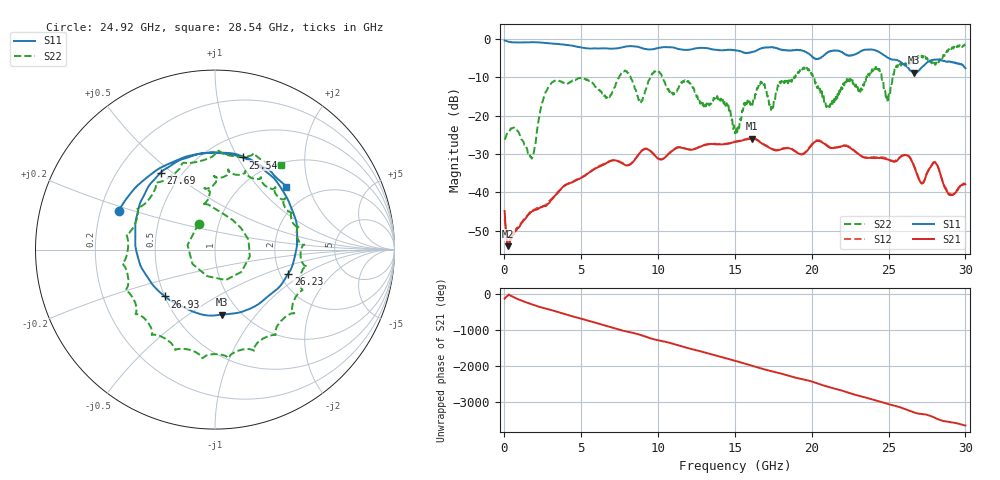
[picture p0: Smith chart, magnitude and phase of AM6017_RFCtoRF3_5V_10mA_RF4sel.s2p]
!Agilent Technologies,E8364B,MY43040894,A.07.50.67
!Agilent E8364B: A.07.50.67
!Date: Tuesday, August 21, 2018 13:40:35
!Correction: S11(Full 2 Port(1,2))
!S21(Full 2 Port(1,2))
!S12(Full 2 Port(1,2))
!S22(Full 2 Port(1,2))
!S2P File: Measurements: S11, S21, S12, S22:
# Hz S  dB  R 50
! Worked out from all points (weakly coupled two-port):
!   1601 points, 10 MHz to 30 GHz, reference 50 ohm
!   highest |S21| = -25.96 dB at 16.13 GHz (marker M1); lowest = -54.0 dB at 234.9 MHz (marker M2)
!   lowest |S11| = -8.8 dB at 26.63 GHz (marker M3), VSWR 2.15, Z = 41.2 - j34.4 ohm
!   |S11| at or under -10 dB: nowhere
!   |S22| runs from -31.2 to -1.3 dB; largest |S21 - S12| = 0.01
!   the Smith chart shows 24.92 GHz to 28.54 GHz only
!   S11 on the Smith chart (normalised r, x): 24.92 GHz: 0.28, +0.18; 25.54 GHz: 0.73, +1.05; 26.23 GHz: 2.21, -0.73; 26.93 GHz: 0.50, -0.31; 27.69 GHz: 0.38, +0.46; 28.54 GHz: 1.48, +1.43
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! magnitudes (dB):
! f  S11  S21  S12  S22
! 10 MHz  -0.3  -44.9  -47.0  -26.2
! 234.9 MHz  -0.6  -54.0  -52.9  -24.2
! 1.772 GHz  -0.8  -45.0  -44.9  -31.2
! 2.897 GHz  -1.0  -42.8  -42.3  -12.2
! 5.015 GHz  -2.2  -36.2  -36.1  -10.1
! 7.882 GHz  -1.9  -32.9  -32.8  -8.3
! 8.857 GHz  -2.2  -29.5  -29.4  -16.7
! 10.02 GHz  -2.3  -31.2  -31.1  -8.5
! 15.01 GHz  -2.8  -26.9  -26.7  -24.5
! 16.13 GHz  -3.4  -26.0  -25.8  -17.2
! 20.01 GHz  -4.5  -27.6  -27.4  -9.3
! 21.06 GHz  -3.4  -28.1  -27.8  -18.0
! 24.17 GHz  -3.0  -31.0  -30.8  -7.2
! 24.92 GHz  -4.8  -31.4  -31.2  -15.3
! 25.01 GHz  -5.0  -31.5  -31.4  -14.3
! 25.54 GHz  -5.4  -31.8  -31.5  -7.1
! 26.23 GHz  -7.3  -30.4  -30.3  -6.2
! 26.63 GHz  -8.8  -32.9  -32.7  -5.7
! 26.93 GHz  -8.4  -36.1  -35.9  -4.4
! 27.69 GHz  -5.6  -33.5  -33.4  -5.9
! 28.54 GHz  -5.6  -37.5  -37.3  -4.5
! 30 GHz  -7.6  -37.9  -37.7  -1.3
